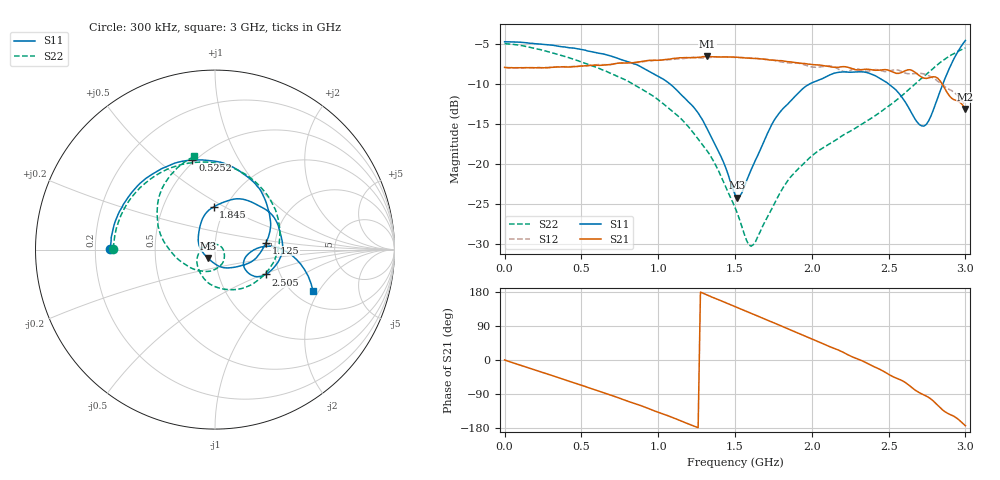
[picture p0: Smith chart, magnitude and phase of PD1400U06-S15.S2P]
!Agilent Technologies,E5071B,MY42302032,A.08.01
!Date: Sat Mar 25 16:48:55 2017
!Data & Calibration Information:
!Freq	S11:SOLT2(ON)	S21:SOLT2(ON)	S12:SOLT2(ON)	S22:SOLT2(ON)
# Hz S dB R 50
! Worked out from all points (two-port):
!   201 points, 300 kHz to 3 GHz, reference 50 ohm
!   highest |S21| = -6.54 dB at 1.32 GHz (marker M1); lowest = -13.1 dB at 3 GHz (marker M2)
!   |S21| within 3 dB of the highest: start of sweep to 2.832 GHz
!   lowest |S11| = -24.2 dB at 1.515 GHz (marker M3), VSWR 1.13, Z = 46 - j4.34 ohm
!   |S11| at or under -10 dB: 1.077 GHz to 1.985 GHz (908.3 MHz wide, 59.3 % of centre); 2.501 GHz to 2.853 GHz (351.9 MHz wide, 13.1 % of centre)
!   |S22| runs from -30.3 to -4.9 dB; largest |S21 - S12| = 0.038
!   S11 on the Smith chart (normalised r, x): 300 kHz: 0.26, +0.00; 525.2 MHz: 0.48, +0.66; 1.125 GHz: 1.79, +0.15; 1.845 GHz: 0.88, +0.44; 2.505 GHz: 1.69, -0.52; 3 GHz: 2.50, -1.78
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300000  -4.70 179.9  -7.91 0.2  -7.92 0.1  -4.92 179.5
1.50285e8  -4.84 157.8  -7.95 -20.1  -7.93 -20.1  -5.32 140.5
2.552745e8  -5.03 142.9  -7.96 -33.8  -7.94 -33.9  -5.80 114.4
3.752625e8  -5.33 125.6  -7.84 -50.0  -7.83 -49.8  -6.45 85.5
5.10249e8  -5.70 106.4  -7.74 -67.9  -7.76 -67.9  -7.31 53.8
5.252475e8  -5.75 104.2  -7.71 -69.9  -7.73 -69.9  -7.41 50.3
7.50225e8  -6.88 70.5  -7.37 -101.1  -7.35 -101.1  -9.15 -2.1
1.0052e9  -9.10 28.6  -7.01 -138.6  -7.00 -139.0  -12.04 -62.9
1.125188e9  -10.84 7.8  -6.75 -156.9  -6.85 -157.1  -13.95 -93.7
1.320168e9  -15.66 -34.0  -6.54 171.3  -6.71 171.7  -18.41 -147.4
1.50015e9  -23.85 -115.7  -6.64 141.1  -6.66 141.2  -25.47 145.9
1.515148e9  -24.24 -130.1  -6.64 138.5  -6.66 138.7  -26.18 138.5
1.60514e9  -20.74 165.1  -6.78 123.2  -6.75 123.1  -30.31 71.7
1.845116e9  -12.48 91.7  -7.20 82.3  -7.34 82.2  -22.07 -52.4
2.010099e9  -9.77 58.8  -7.57 54.2  -7.89 54.3  -18.86 -94.0
2.29507e9  -8.46 7.0  -8.23 3.2  -8.09 5.2  -15.40 -143.5
2.50505e9  -10.06 -26.1  -8.29 -38.9  -8.36 -35.2  -12.69 -172.6
2.640036e9  -13.30 -34.6  -8.21 -68.9  -8.71 -66.5  -10.53 168.8
2.730027e9  -15.27 -17.8  -9.26 -92.1  -8.74 -89.8  -9.04 154.7
2.80502e9  -12.53 1.9  -9.11 -113.6  -9.42 -112.0  -7.79 141.7
2.880012e9  -8.72 0.8  -11.03 -139.7  -10.52 -132.9  -6.70 127.4
3e9  -4.54 -22.9  -13.13 -173.4  -12.60 -171.1  -5.49 102.7
